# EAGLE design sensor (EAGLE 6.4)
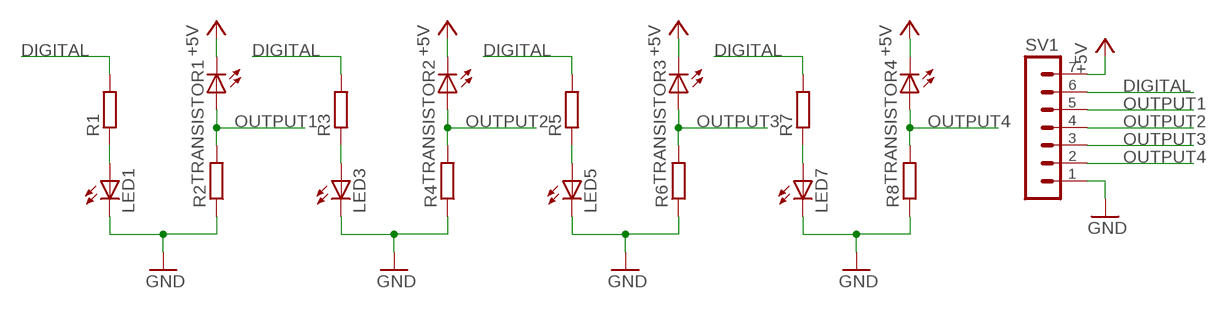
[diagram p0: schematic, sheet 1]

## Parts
LED1  LED5MM  [LED5MM]
LED3  LED5MM  [LED5MM]
LED5  LED5MM  [LED5MM]
LED7  LED5MM  [LED5MM]
R1  R-EU_0207/12  [0207/12]
R2  R-EU_0207/12  [0207/12]
R3  R-EU_0207/12  [0207/12]
R4  R-EU_0207/12  [0207/12]
R5  R-EU_0207/12  [0207/12]
R6  R-EU_0207/12  [0207/12]
R7  R-EU_0207/12  [0207/12]
R8  R-EU_0207/12  [0207/12]
SV1  MA07-1  [MA07-1]
TRANSISTOR1  LED5MM  [LED5MM]
TRANSISTOR2  LED5MM  [LED5MM]
TRANSISTOR3  LED5MM  [LED5MM]
TRANSISTOR4  LED5MM  [LED5MM]

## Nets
+5V: SV1.7 TRANSISTOR1.K(C) TRANSISTOR2.K(C) TRANSISTOR3.K(C) TRANSISTOR4.K(C)
DIGITAL: R1.2 R3.2 R5.2 R7.2 SV1.6
GND: LED1.K(C) LED3.K(C) LED5.K(C) LED7.K(C) R2.1 R4.1 R6.1 R8.1 SV1.1
N$1: LED3.A R3.1
N$3: LED1.A R1.1
N$5: LED5.A R5.1
N$7: LED7.A R7.1
OUTPUT1: R2.2 SV1.5 TRANSISTOR1.A
OUTPUT2: R4.2 SV1.4 TRANSISTOR2.A
OUTPUT3: R6.2 SV1.3 TRANSISTOR3.A
OUTPUT4: R8.2 SV1.2 TRANSISTOR4.A

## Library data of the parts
LED1 LED3 LED5 LED7 TRANSISTOR1-TRANSISTOR4 = led:LED: LED
R1-R8 = rcl:R-EU_: RESISTOR, European symbol
SV1 = con-lstb:MA07-1: PIN HEADER; OC_FARNELL: unknown; OC_NEWARK: unknown

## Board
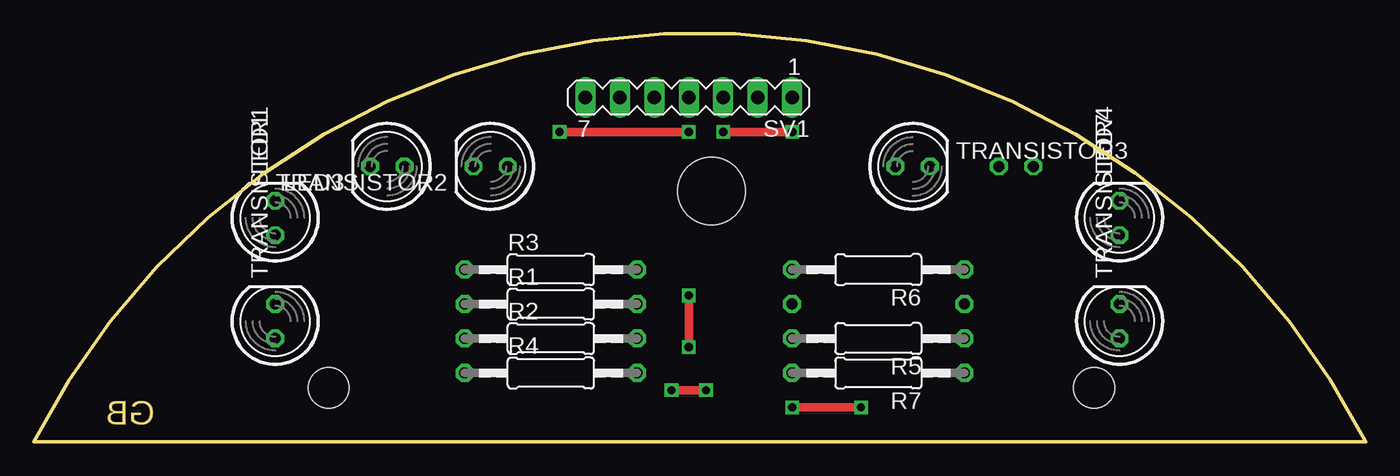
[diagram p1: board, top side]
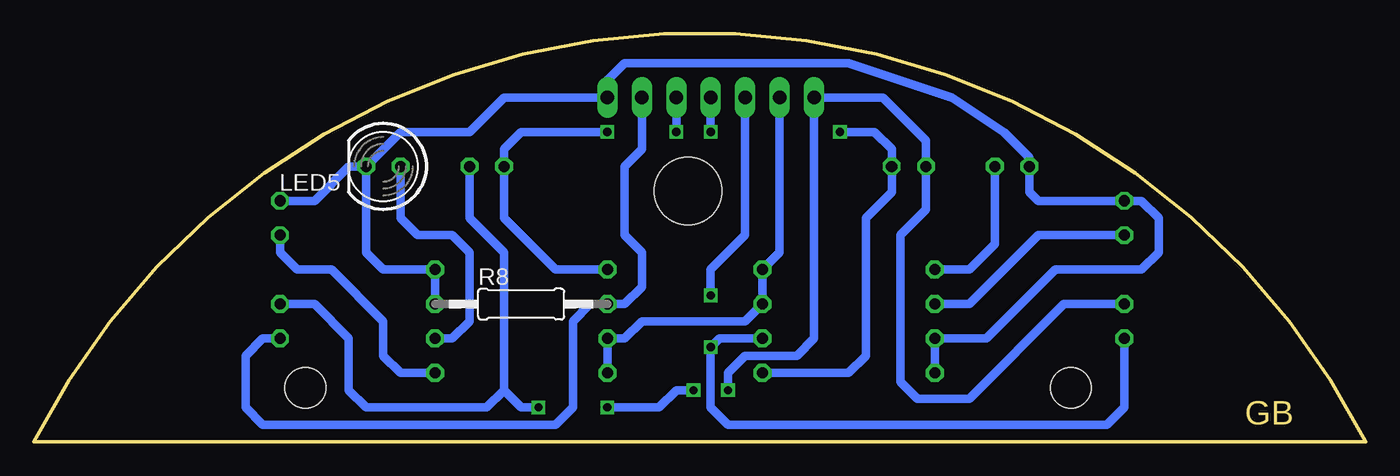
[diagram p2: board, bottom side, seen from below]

Size 98.14 x 30.09 mm. Coordinates in mm from the lower left corner, seen from the top.
Outline: 98.14,0 0,0 arc-126 98.14,0
Copper layers (1*16): Top 0.035mm / dielectric 1.5mm / Bottom 0.035mm
Design rules "default": minimum track width 10mil, minimum drill 24mil, track to track 8mil, track to pad 8mil, pad to pad 8mil, via to via 8mil, smd to smd 8mil, copper to edge 40mil, drill to drill 8mil, minimum pad ring 10mil, minimum via ring 8mil, stop-mask expansion 4mil, vias tented up to drill 0mil, thermal gap 10mil
Holes 3 mm at 78.13,3.98 21.73,3.98
Holes 5 mm at 49.93,18.49

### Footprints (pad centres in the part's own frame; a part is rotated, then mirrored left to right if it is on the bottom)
LED5MM = drill 0.813 octagon: A -1.27,0; K 1.27,0
0207/12 = drill 0.813 octagon: 1 -6.35,0; 2 6.35,0
MA07-1 = drill 1.016 long: 1 -7.62,0; 2 -5.08,0; 3 -2.54,0; 4 0,0; 5 2.54,0; 6 5.08,0; 7 7.62,0

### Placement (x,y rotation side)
LED1  17.78,16.51 90 top
LED3  26.04,20.32 180 top
LED5  72.39,20.32 180 bottom
LED7  80.01,16.51 90 top
R1  38.1,10.16 0 top
R2  38.1,7.62 0 top
R3  38.1,12.7 0 top
R4  38.1,5.08 0 top
R5  62.23,7.62 180 top
R6  62.23,12.7 180 top
R7  62.23,5.08 180 top
R8  62.23,10.16 0 bottom
SV1  48.26,25.4 180 top
TRANSISTOR1  17.78,8.89 90 top
TRANSISTOR2  33.66,20.32 180 top
TRANSISTOR3  64.77,20.32 0 top
TRANSISTOR4  80.01,8.89 90 top

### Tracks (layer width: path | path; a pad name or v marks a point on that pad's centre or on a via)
+5V  (via drill 0.6)
  Top 0.61: v46.99,3.81 v49.53,3.81 | v55.88,2.54 v60.96,2.54
  Bottom 0.61: TRANSISTOR4.K 77.47,10.16 74.93,7.62 74.93,3.81 73.66,2.54 64.77,2.54 63.5,3.81 | TRANSISTOR1.K 22.23,10.16 29.21,3.17 33.02,3.17 34.29,4.45 34.29,15.24 32.38,17.14 TRANSISTOR2.K 32.38,22.23 35.56,25.4 SV1.7 40.64,7.62 41.91,6.35 45.72,6.35 46.99,5.08 v46.99,3.81 | TRANSISTOR3.K 66.04,16.51 63.5,13.97 63.5,3.81 | v49.53,3.81 50.8,3.81 52.07,2.54 v55.88,2.54 | v60.96,2.54 62.23,2.54 63.5,3.81
DIGITAL
  Bottom 0.61: R7.2 R5.2 54.61,7.62 53.34,8.89 45.72,8.89 R1.2 R3.2 43.18,13.97 SV1.6
GND
  Bottom 0.406: LED3.K 24.77,20.95
  Bottom 0.61: R8.1 R6.1 72.39,12.7 73.66,13.97 LED5.K | R4.1 R2.1 27.94,7.62 22.86,12.7 16.51,12.7 15.24,13.97 15.24,16.51 16.51,17.78 LED1.K 24.13,17.78 24.77,18.41 LED3.K | LED5.K 71.12,22.86 66.04,22.86 63.5,25.4 SV1.1 55.88,26.67 54.61,27.94 38.1,27.94 30.48,25.4 26.67,22.86 24.77,20.95 | LED7.K 77.47,17.78 74.93,20.32 LED5.K
N$1
  Bottom 0.61: LED3.A 27.3,14.61 29.21,12.7 R3.1
N$3
  Bottom 0.61: LED1.A 24.13,15.24 29.21,10.16 R1.1
N$5
  Bottom 0.61: R5.1 67.31,7.62 66.04,8.89 66.04,13.97 67.31,15.24 69.85,15.24 71.12,16.51 LED5.A
N$7
  Bottom 0.61: R7.1 71.12,5.08 72.39,6.35 72.39,8.89 76.2,12.7 78.74,12.7 80.01,13.97 LED7.A
OUTPUT1  (via drill 0.6)
  Top 0.61: v48.26,10.79 v48.26,6.99
  Bottom 0.61: TRANSISTOR1.A 17.78,2.54 19.05,1.27 46.99,1.27 48.26,2.54 v48.26,6.99 47.62,7.62 R2.2 | SV1.5 45.72,15.24 48.26,12.7 v48.26,10.79
OUTPUT2  (via drill 0.6)
  Top 0.61: v48.26,22.86 v38.73,22.86
  Bottom 0.61: R4.2 38.1,5.08 36.83,6.35 36.83,16.51 34.92,18.41 TRANSISTOR2.A 34.92,21.59 36.2,22.86 v38.73,22.86 | SV1.4 v48.26,22.86
OUTPUT3  (via drill 0.6)
  Top 0.61: v50.8,22.86 v55.88,22.86
  Bottom 0.61: R6.2 59.69,12.7 63.5,16.51 TRANSISTOR3.A 63.5,21.59 62.23,22.86 v55.88,22.86 | SV1.3 v50.8,22.86
OUTPUT4
  Bottom 0.61: TRANSISTOR4.A 81.28,7.62 82.55,6.35 82.55,2.54 81.28,1.27 59.69,1.27 58.42,2.54 58.42,8.89 57.15,10.16 R8.2 54.61,10.16 53.34,11.43 53.34,13.97 54.61,15.24 54.61,20.32 53.34,21.59 SV1.2

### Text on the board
Dimension: GB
